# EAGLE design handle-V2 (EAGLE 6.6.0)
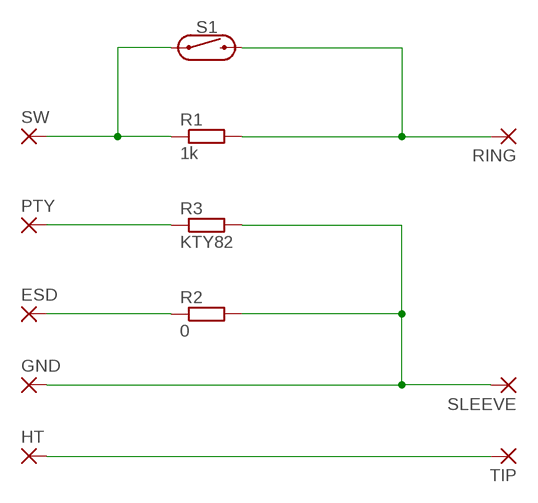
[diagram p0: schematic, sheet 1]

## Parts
ESD  SMD2  [SMD1,27-2,54]
GND  WIREPADSMD5-1,8  [5-1,8]
HT  WIREPADSMD5-1,8  [5-1,8]
PTY  SMD2  [SMD1,27-2,54]
R1  1k  R-EU_R0805  [R0805]
R2  0  R-EU_R0805  [R0805]
R3  KTY82  R-EU_R0805  [R0805]
RING  WIREPADSMD5-1,8  [5-1,8]
S1  REED_SWITCH-PTH-INSULATED  [REED_SWITCH_PLASTIC]
SLEEVE  WIREPADSMD5-1,8  [5-1,8]
SW  SMD2  [SMD1,27-2,54]
TIP  WIREPADSMD5-1,8  [5-1,8]

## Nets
ESD: ESD.1(P) R2.1
GND: GND.1(P) R2.2 R3.2 SLEEVE.1(P)
HEATHER: HT.1(P) TIP.1(P)
N$2: R1.2 RING.1(P) S1.P$2
PTC: PTY.1(P) R3.1
SW: R1.1 S1.P$1 SW.1(P)

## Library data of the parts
ESD PTY SW = wirepad:SMD2: SMD PAD
GND HT RING SLEEVE TIP = wirepad:WIREPAD: Wire PAD connect wire on PCB
R1-R3 = resistor:R-EU_: RESISTOR, European symbol
S1 = SparkFun-Switches:REED_SWITCH: Reed Switch; PROD_ID: SWCH-10467; SF_SKU: COM-10601

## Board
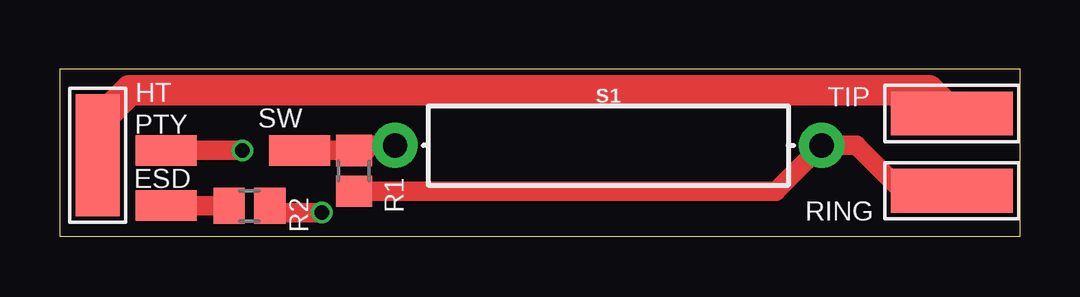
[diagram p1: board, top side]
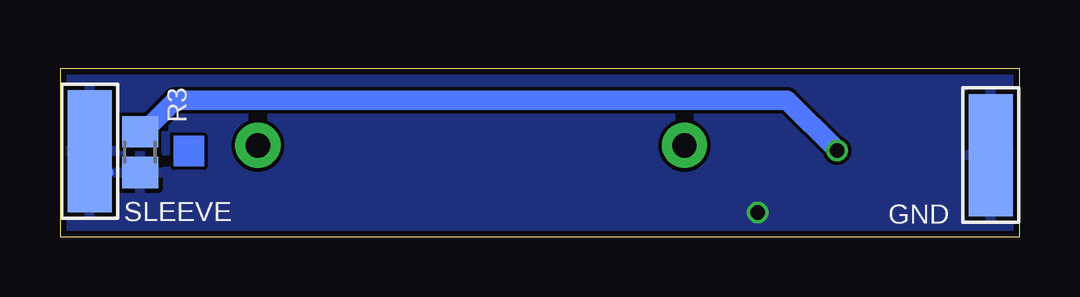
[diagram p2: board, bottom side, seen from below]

Size 40 x 7 mm. Coordinates in mm from the lower left corner, seen from the top.
Outline: 0,0 0,7 40,7 40,0 0,0
Copper layers (1*16): Top 0.018mm / dielectric 1.55mm / Bottom 0.018mm
Design rules "rdy_default": minimum track width 0.15mm, minimum drill 0.35mm, track to track 0.15mm, track to pad 0.15mm, pad to pad 0.15mm, via to via 0.15mm, smd to smd 0mil, copper to edge 0.25mm, drill to drill 0.35mm, minimum pad ring 0.175mm, minimum via ring 0.125mm, stop-mask expansion 0mil, vias tented up to drill 0.45mm, thermal gap 0.2mm

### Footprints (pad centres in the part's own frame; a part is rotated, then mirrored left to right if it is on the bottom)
SMD1,27-2,54 = smd 1.27 x 2.54: 1 0,0
5-1,8 = smd 1.829 x 5.08: 1 0,0
R0805 = smd 1.3 x 1.5: 1 -0.85,0; 2 0.85,0
REED_SWITCH_PLASTIC = drill 1.016 pad 1.88: P$1 -8.89,0; P$2 8.89,0

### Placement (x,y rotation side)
ESD  4.43,1.3 270 top
GND  1.19,3.41 180 bottom
HT  1.57,3.4 180 top
PTY  4.43,3.6 270 top
R1  12.25,2.75 270 top
R2  7.9,1.29 0 top
R3  36.66,3.53 270 bottom
RING  37.17,1.92 90 top
S1  22.86,3.81 0 top
SLEEVE  38.76,3.56 180 bottom
SW  9.98,3.6 270 top
TIP  37.18,5.14 90 top

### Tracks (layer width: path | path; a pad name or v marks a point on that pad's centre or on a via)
ESD
  Top 0.813: R2.1 ESD.1
GND  (via drill 0.6)
  Top 0.813: v10.92,1.01 9.03,1.01 R2.2
  Bottom 0.406: 37.96,2.68 38.1,2.54 38.1,2.9 SLEEVE.1
  pour Bottom: 0.2,6.8 39.8,6.8 39.8,0.2 0.2,0.2
HEATHER
  Top 1.27: HT.1 1.57,4.77 2.9,6.1 36.22,6.1 TIP.1
N$2
  Top 0.813: RING.1 37.09,2 35,2 33.19,3.81 S1.P$2 29.84,1.9 R1.2
PTC  (via drill 0.6)
  Top 0.813: v7.6,3.6 PTY.1
  Bottom 0.813: R3.1 36.52,4.38 35.2,5.7 9.7,5.7 v7.6,3.6
SW
  Top 0.813: 12.96,3.81 12.72,3.74 | 12.72,3.74 R1.1 | 12.75,3.6 R1.1 | SW.1 R1.1 | S1.P$1 12.72,3.81 12.72,3.74
(copper drawn outside any net)
  shapes: Bottom area x1

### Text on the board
Reference: Weller_Handle_V2
_tNames: HT | S1 | TIP | SW | PTY | R3 | ESD | R1 | RING | R2
_bNames: GND | SLEEVE

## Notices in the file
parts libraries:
SparkFun-Switches: Licensing: Creative Commons ShareAlike 4.0 International - https://creativecommons.org/licenses/by-sa/4.0
